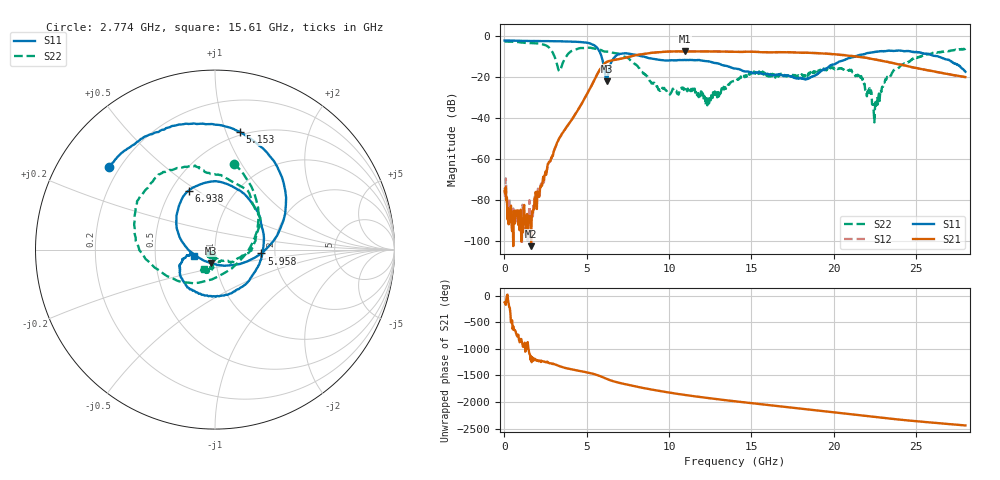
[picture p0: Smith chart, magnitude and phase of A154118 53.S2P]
!  2-Port S-parameters saved by WinCal
! VAR MeasName=S-Parameters (CALIBRATED_DATA) read from VNA (N5230A)
! VAR MeasDate=2015-9-10 14:39:15
! VAR NAME=A154118 53
! VAR FILENAME=A154118 53.S2P
! VAR DATE=2015-9-10 14:39:15
! VAR PHYS_PORTS=1,2
# Hz S DB R 50
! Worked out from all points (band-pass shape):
!   801 points, 10 MHz to 28 GHz, reference 50 ohm
!   highest |S21| = -7.45 dB at 10.96 GHz (marker M1); lowest = -102.3 dB at 1.619 GHz (marker M2)
!   |S21| within 3 dB of the highest: 7.405 GHz to 21.86 GHz (14.45 GHz wide, 98.8 % of centre)
!   lowest |S11| = -22.1 dB at 6.203 GHz (marker M3), VSWR 1.17, Z = 47.1 - j7.05 ohm
!   |S11| at or under -10 dB: 5.897 GHz to 6.723 GHz (825.6 MHz wide, 13.1 % of centre); 8.459 GHz to 21.32 GHz (12.86 GHz wide, 86.4 % of centre); 26.38 GHz to end of sweep
!   |S22| runs from -42.0 to -2.7 dB; largest |S21 - S12| = 0.0092
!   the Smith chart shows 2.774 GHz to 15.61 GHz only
!   S11 on the Smith chart (normalised r, x): 2.774 GHz: 0.16, +0.34; 5.153 GHz: 0.47, +1.12; 5.958 GHz: 1.70, -0.08; 6.938 GHz: 0.61, +0.46; 15.61 GHz: 0.79, -0.06
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1e7  -2.15 179.7  -75.61 -125.5  -73.88 -143.3  -2.67 179.8
1.619425e9  -2.42 158.7  -102.31 -61.3  -90.09 -76.4  -3.43 141.2
2.774012e9  -2.49 142.1  -61.04 167.4  -61.10 162.9  -6.22 77.8
3.543738e9  -2.61 128.2  -47.07 92.5  -46.96 93.6  -13.05 -122.7
4.698325e9  -3.01 98.3  -32.89 16.3  -32.89 16.2  -5.83 145.0
5.153162e9  -3.48 78.0  -26.23 -13.2  -26.21 -13.1  -5.66 126.2
5.957875e9  -11.71 -4.8  -14.44 -92.6  -14.39 -92.5  -7.19 97.5
6.202788e9  -22.11 -108.5  -12.68 -125.3  -12.63 -125.5  -7.59 88.1
6.937525e9  -8.88 114.2  -11.26 162.8  -11.23 162.5  -8.64 59.4
8.1271e9  -9.45 54.8  -9.11 82.0  -9.10 81.8  -15.11 -7.2
9.351662e9  -11.54 -4.6  -7.91 10.9  -7.85 10.7  -26.15 -82.1
1.096109e10  -11.68 -90.0  -7.45 -67.6  -7.40 -68.2  -25.94 -129.1
1.236059e10  -12.27 -142.4  -7.51 -125.7  -7.45 -126.3  -29.72 -137.2
1.4005e10  -15.83 -167.9  -7.69 172.7  -7.66 172.1  -21.64 -100.2
1.561442e10  -18.28 -161.6  -7.87 115.9  -7.86 115.0  -18.05 -119.7
1.869332e10  -19.58 -113.8  -8.22 10.6  -8.23 10.1  -17.13 -111.1
2.103749e10  -10.41 -114.1  -9.74 -72.2  -9.64 -73.2  -16.79 -156.4
2.166726e10  -9.01 -121.3  -10.28 -94.1  -10.22 -95.4  -19.48 -169.0
2.247198e10  -7.72 -135.9  -11.34 -122.8  -11.31 -123.9  -42.04 -14.7
2.334666e10  -7.15 -150.2  -12.76 -151.6  -12.70 -153.3  -19.62 -19.6
2.495609e10  -7.72 -177.7  -15.47 160.1  -15.49 158.8  -10.85 -58.8
2.8e10  -17.37 134.4  -19.99 78.1  -20.05 77.3  -6.09 -102.8
